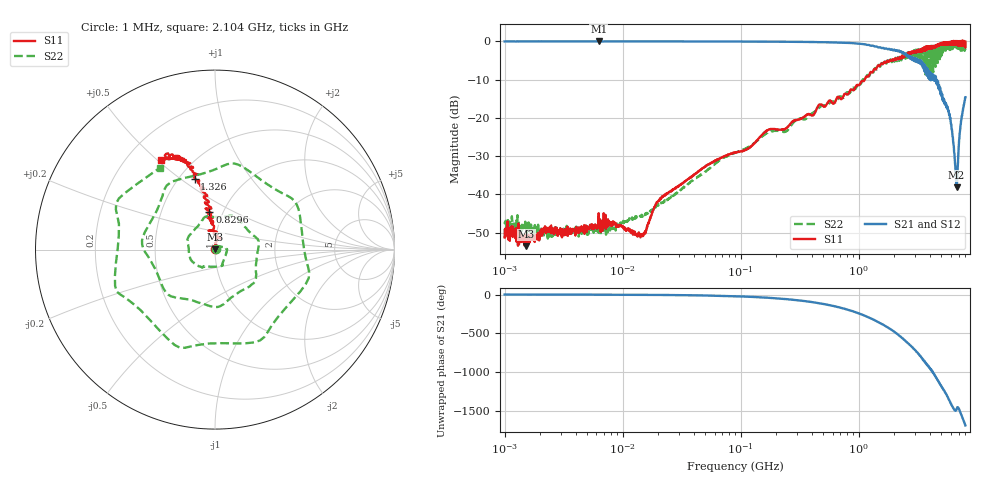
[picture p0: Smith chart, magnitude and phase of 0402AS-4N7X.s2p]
!s-Parameter Generated by FASTRON Sdn. Bhd.
!FASTRON P/N : 0402AS-4N7X
!Keysight Technologies: E5071C_MY46733604_B.14.02
!Date: Mon Dec 01 10:24:15 2025
!Version  :Rev00  Mon Dec 01 10:24:15 2025
!Data & Calibration Information:
!Freq  S11:SOLT2(ON)  S21:SOLT2(ON)  S12:SOLT2(ON)  S22:SOLT2(ON)
!PortZ  Port1:50+j0  Port2:50+j0
!When reading reference impedance value at option line is always used.
! Remarks : This data is being provided solely for informational purposes.
# Hz S dB R 50
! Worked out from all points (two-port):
!   1601 points, 1 MHz to 8 GHz, reference 50 ohm
!   highest |S21| = 0.02 dB at 6.268 MHz (marker M1); lowest = -38.1 dB at 6.728 GHz (marker M2)
!   |S21| within 3 dB of the highest: start of sweep to 2.319 GHz; 2.359 GHz to 2.395 GHz (36.14 MHz wide, 1.52 % of centre)
!   lowest |S11| = -53.5 dB at 1.523 MHz (marker M3), VSWR 1.00, Z = 50.2 + j0.0873 ohm
!   |S11| at or under -10 dB: start of sweep to 1.124 GHz
!   |S22| runs from -51.5 to -0.6 dB; largest |S21 - S12| = 0.016
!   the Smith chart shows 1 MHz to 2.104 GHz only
!   S11 on the Smith chart (normalised r, x): 1 MHz: 1.01, +0.00; 829.6 MHz: 0.86, +0.38; 1.326 GHz: 0.60, +0.57; 2.104 GHz: 0.34, +0.52
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1000000  -51.20 23.7  -0.05 -0.2  -0.01 -0.3  -47.70 27.2
1522827  -53.50 24.3  -0.04 -0.4  -0.03 -0.4  -48.10 -6.7
4479405  -48.30 26.8  -0.05 -1.2  -0.03 -1.1  -50.20 31.3
6268472  -44.90 11.8  0.02 -1.8  0.03 -1.7  -50.00 10.4
2.00676e7  -41.70 39.0  -0.05 -5.0  -0.04 -5.0  -42.90 64.7
8.994653e7  -29.00 90.0  -0.08 -22.2  -0.07 -22.1  -29.10 26.1
4.006501e8  -19.30 104.0  -0.20 -97.5  -0.19 -97.5  -18.90 -124.0
8.295903e8  -13.40 98.4  -0.44 158.0  -0.43 158.0  -13.60 40.4
1.326347e9  -7.72 106.0  -1.20 37.2  -1.19 37.2  -8.17 146.0
1.7949e9  -5.39 111.0  -1.98 -72.8  -1.98 -72.8  -5.47 -78.8
2.103821e9  -4.68 121.0  -2.34 -147.0  -2.32 -147.0  -5.20 124.0
2.340174e9  -3.82 122.0  -3.12 156.0  -3.10 156.0  -3.68 9.3
2.545586e9  -3.47 124.0  -3.72 107.0  -3.68 107.0  -3.07 -89.5
2.736325e9  -2.96 127.0  -4.49 63.0  -4.45 62.9  -2.60 176.0
2.956409e9  -2.96 132.0  -4.46 12.9  -4.42 12.7  -3.07 75.4
3.26428e9  -2.82 140.0  -4.90 -64.8  -4.86 -65.1  -5.00 -84.6
3.60885e9  -1.97 148.0  -7.16 -140.0  -7.13 -141.0  -1.93 98.1
4.014226e9  -1.98 152.0  -8.08 128.0  -8.08 127.0  -1.34 -87.2
4.352635e9  -1.22 156.0  -10.30 47.6  -10.40 47.1  -6.43 132.0
5.500301e9  -0.90 -166.0  -16.70 149.0  -16.70 149.0  -0.89 -79.7
6.72769e9  0.06 -120.0  -38.10 -44.1  -38.10 -43.3  -1.57 53.6
8e9  -0.14 -93.7  -14.60 108.0  -14.50 107.0  -2.32 147.0
